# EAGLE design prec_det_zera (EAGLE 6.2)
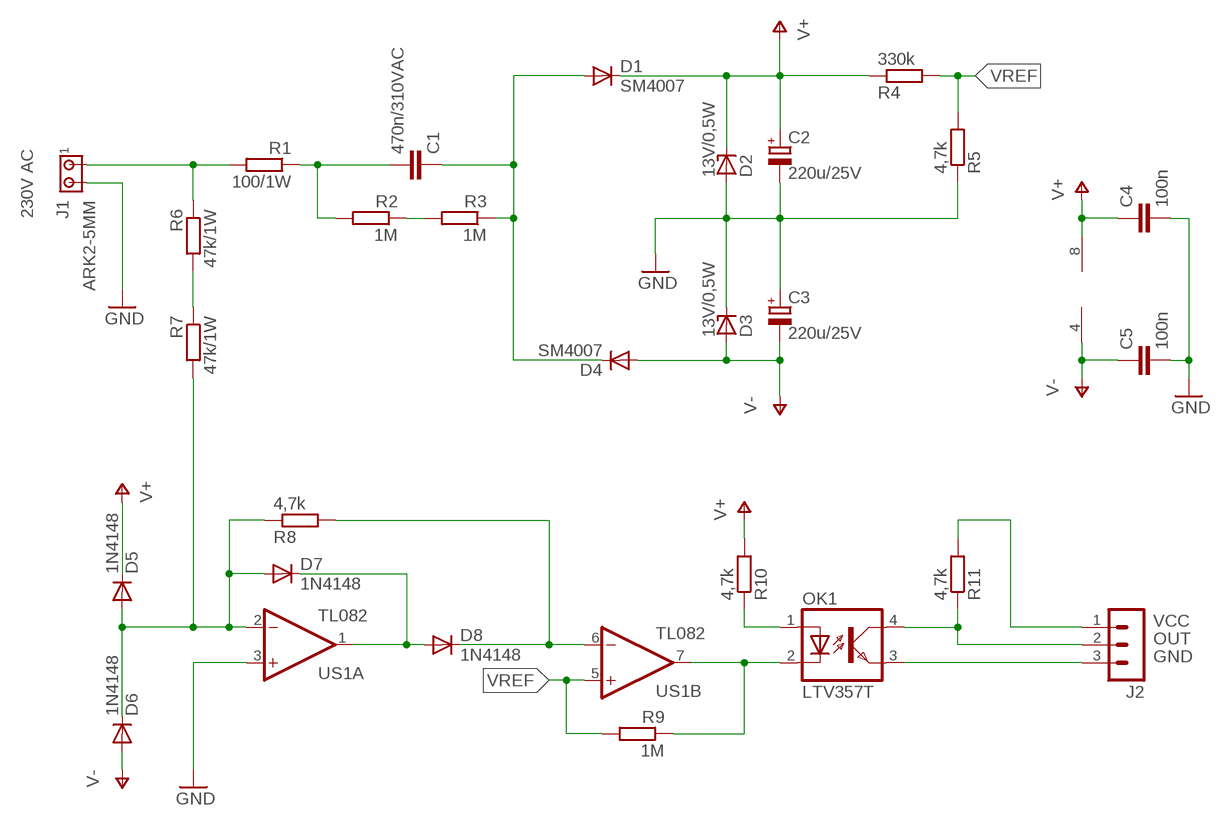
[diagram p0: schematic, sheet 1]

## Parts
C1  470n/310VAC  C-EU225-108X268  [C225-108X268]
C2  220u/25V  CPOL-EUE3.5-8  [E3,5-8]
C3  220u/25V  CPOL-EUE3.5-8  [E3,5-8]
C4  100n  C-EUC0805  [C0805]
C5  100n  C-EUC0805  [C0805]
D1  SM4007  DIODE-MELF-MLL41  [MELF-MLL41]
D2  13V/0,5W  ZENER-DIODESOD80C  [SOD80C]
D3  13V/0,5W  ZENER-DIODESOD80C  [SOD80C]
D4  SM4007  DIODE-MELF-MLL41  [MELF-MLL41]
D5  1N4148  DIODE-MINIMELF  [MINIMELF]
D6  1N4148  DIODE-MINIMELF  [MINIMELF]
D7  1N4148  DIODE-MINIMELF  [MINIMELF]
D8  1N4148  DIODE-MINIMELF  [MINIMELF]
J1  ARK2-5MM  [2PIN-5MM]
J2  MA03-1  [MA03-1]
OK1  LTV357T  SFH6186-3  [SMD4-7]
R1  100/1W  R-EU_0411/12  [0411/12]
R2  1M  R-EU_M0805  [M0805]
R3  1M  R-EU_M0805  [M0805]
R4  330k  R-EU_M0805  [M0805]
R5  4,7k  R-EU_M0805  [M0805]
R6  47k/1W  R-EU_0411/12  [0411/12]
R7  47k/1W  R-EU_0411/12  [0411/12]
R8  4,7k  R-EU_M0805  [M0805]
R9  1M  R-EU_M0805  [M0805]
R10  4,7k  R-EU_M0805  [M0805]
R11  4,7k  R-EU_M0805  [M0805]
US1  TL082  TL082D  [SO08]

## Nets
+15V: C2.+ C4.1 D1.C D2.C D5.C R4.1 R10.2 US1.8(P:V+) ; supply symbol labelled V+
-15V: C3.- C5.1 D3.A D4.A D6.A US1.4(P:V-) ; supply symbol labelled V-
GND: C2.- C3.+ C4.2 C5.2 D2.A D3.C J1.P$2 R5.1 US1.3(A:+IN)
N$1: OK1.2(C) R9.1 US1.7(B:OUT)
N$2: D5.A D6.C D7.A R7.2 R8.1 US1.2(A:-IN)
N$3: R6.2 R7.1
N$4: D7.C D8.A US1.1(A:OUT)
N$5: D8.C R8.2 US1.6(B:-IN)
N$6: OK1.1(A) R10.1
N$7: J2.3 OK1.3(EMIT)
N$8: J1.P$1 R1.2 R6.1
N$9: J2.2 OK1.4(COL) R11.1
N$10: J2.1 R11.2
N$17: C1.2 R1.1 R2.2
N$19: R2.1 R3.2
N$20: C1.1 D1.A D4.C R3.1
VREF: R4.2 R5.2 R9.2 US1.5(B:+IN)

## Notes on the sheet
- 230V AC
- VCC
- OUT
- GND

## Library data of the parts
C1 C4 C5 = rcl:C-EU: CAPACITOR, European symbol
C2 C3 = rcl:CPOL-EU: POLARIZED CAPACITOR, European symbol
D1 D4-D8 = diode:DIODE-: DIODE
D2 D3 = diode:ZENER-DIODE: Z-Diode
J1 = zlacza_futrzak:ARK2: ARK 2
J2 = con-lstb:MA03-1: PIN HEADER; OC_FARNELL: unknown; OC_NEWARK: unknown
OK1 = optocoupler:SFH618?*: Optocoupler, Phototransistor Output, Low Input Current Source: Data sheet; MF: VISHAY/TELEFUNKEN; MPN: SFH6186-3; OC_FARNELL: 1469529; OC_NEWARK: 21H7751
R1-R11 = rcl:R-EU_: RESISTOR, European symbol
US1 = linear:TL082: OP AMP

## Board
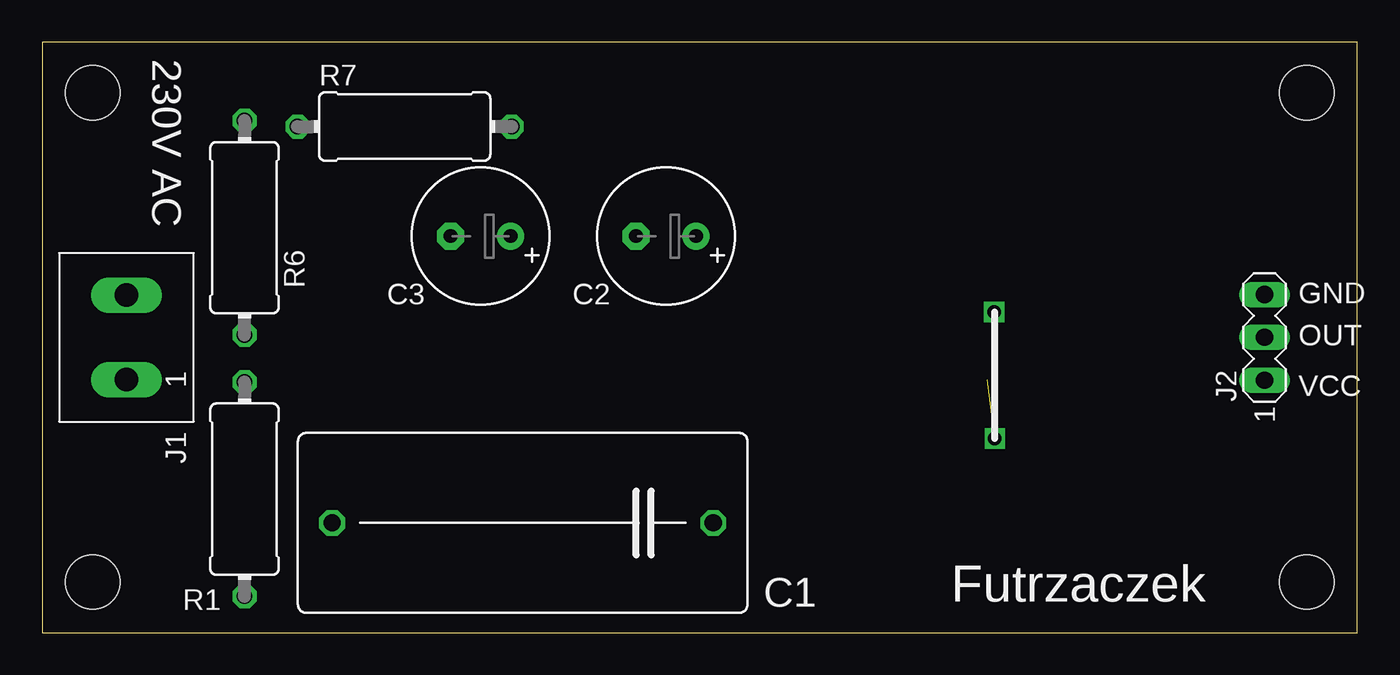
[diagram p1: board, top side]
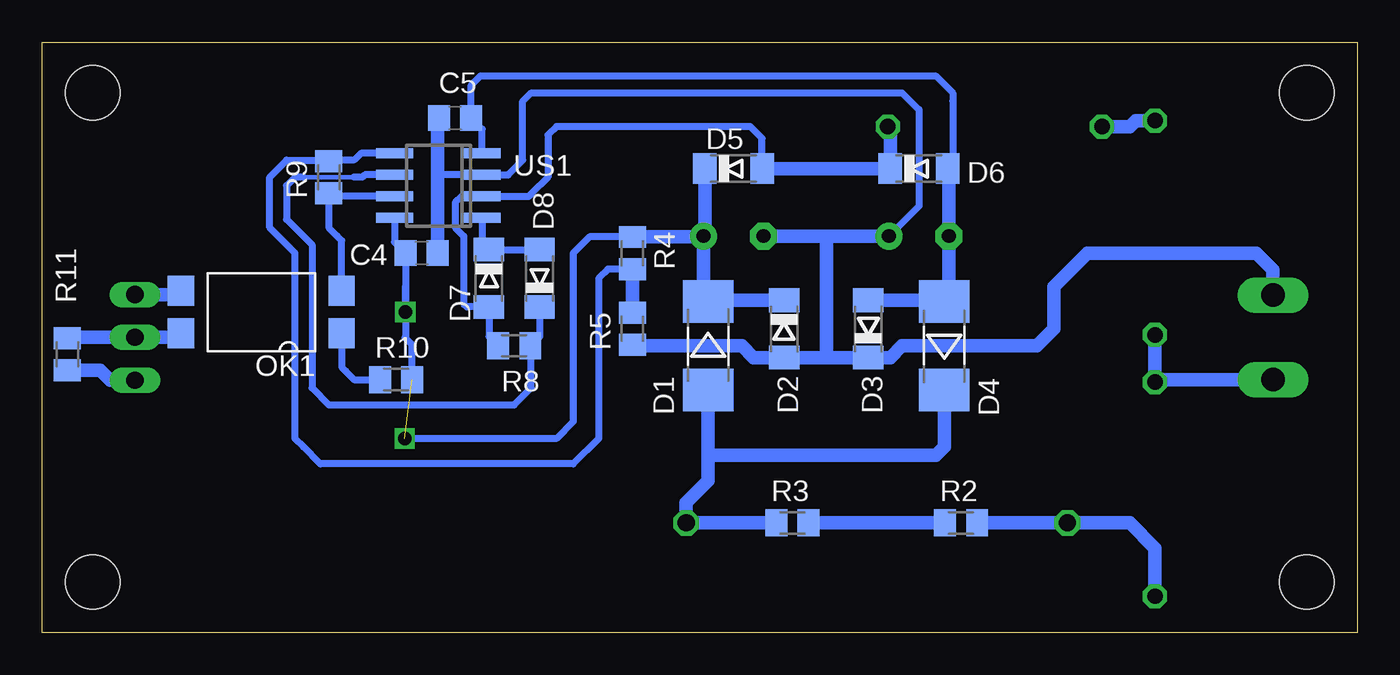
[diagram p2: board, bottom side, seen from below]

Size 78 x 35 mm. Coordinates in mm from the lower left corner, seen from the top.
Outline: 0,0 78,0 78,35 0,35 0,0
Copper layers (1*16): Top 0.035mm / dielectric 1.5mm / Bottom 0.035mm
Design rules: minimum track width 10mil, minimum drill 24mil, track to track 8mil, track to pad 8mil, pad to pad 8mil, via to via 8mil, smd to smd 8mil, copper to edge 40mil, drill to drill 8mil, minimum pad ring 10mil, minimum via ring 8mil, stop-mask expansion 4mil, vias tented up to drill 0mil, thermal gap 10mil
Holes 3.2 mm at 3,3 3,32 75,3 75,32

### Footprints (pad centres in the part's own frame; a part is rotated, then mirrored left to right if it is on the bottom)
C225-108X268 = drill 1.016 octagon: 1 -11.303,0; 2 11.303,0
E3,5-8 = drill 0.813 pad 1.6: + -1.778,0 | drill 0.813 pad 1.6 octagon: - 1.778,0
C0805 = smd 1.3 x 1.5: 1 -0.95,0; 2 0.95,0
MELF-MLL41 = smd 2.5 x 3: A 2.625,0; C -2.625,0
SOD80C = smd 1.4 x 1.8: A 1.7,0; C -1.7,0
MINIMELF = smd 1.4 x 1.8: A 1.7,0; C -1.7,0
2PIN-5MM = drill 1.4 long: P$1 -2.5,0; P$2 2.5,0
MA03-1 = drill 1.016 long: 1 -2.54,0; 2 0,0; 3 2.54,0
SMD4-7 = smd 1.78 x 1.55: 1 -1.27,-4.77; 2 1.27,-4.77; 3 1.27,4.77; 4 -1.27,4.77
0411/12 = drill 0.914 octagon: 1 -6.35,0; 2 6.35,0
M0805 = smd 1.3 x 1.6: 1 -0.95,0; 2 0.95,0
SO08 = smd 0.6 x 2.2: 1 -1.905,-2.6; 2 -0.635,-2.6; 3 0.635,-2.6; 4 1.905,-2.6; 5 1.905,2.6; 6 0.635,2.6; 7 -0.635,2.6; 8 -1.905,2.6

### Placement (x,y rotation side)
C1  28.5,6.5 180 top
C2  37,23.5 180 top
C3  26,23.5 180 top
C4  55.5,22.5 0 bottom
C5  53.5,30.5 180 bottom
D1  38.5,17 270 bottom
D2  34,18 270 bottom
D3  29,18 90 bottom
D4  24.5,17 90 bottom
D5  37,27.5 0 bottom
D6  26,27.5 0 bottom
D7  51.5,21 270 bottom
D8  48.5,21 90 bottom
J1  5,17.5 90 top
J2  72.5,17.5 90 top
OK1  65,19 90 bottom
R1  12,8.5 90 top
R2  23.5,6.5 0 bottom
R3  33.5,6.5 0 bottom
R4  43,22.5 270 bottom
R5  43,18 90 bottom
R6  12,24 90 top
R7  21.5,30 0 top
R8  50,17 0 bottom
R9  61,27 90 bottom
R10  57,15 0 bottom
R11  76.5,16.5 270 bottom
US1  54.5,26.5 90 bottom

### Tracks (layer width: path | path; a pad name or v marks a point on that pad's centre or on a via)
+15V  (via drill 0.8)  (1 unrouted)
  Bottom 0.406: US1.8 57.1,23.15 C4.1 56.45,20.5 | 56.45,20.5 v56.45,19 | v56.45,19 56.45,17.55 56.5,17.5 56.05,17.05 R10.2 | R4.1 45.55,23.45 46.5,22.5 46.5,12.5 47.5,11.5 v56.5,11.5 | v56.45,19 56.45,20.5
  Bottom 0.813: D2.C 38.42,19.7 D1.C 38.78,19.9 C2.+ | D5.C 38.7,23.58 C2.+ | R4.1 38.83,23.45 C2.+
-15V
  Bottom 0.406: D6.A 24,27.8 24,31.5 24,32 25,33 52,33 52.55,32.45 C5.1 51.9,29.85 US1.4
  Bottom 0.813: D3.A 24.57,19.7 D4.A 24.22,19.9 C3.- 24.22,27.92 D6.A
GND
  Bottom 0.406: 54.55,27 54.41,27.14 US1.3 50.37,27.14 50,27.5 49.5,28 49.5,31.5 49,32 27,32 26,31 26,25.28 C3.+
  Bottom 0.813: 31.5,16.3 D2.A 35.8,16.3 36.5,17 42.95,17 R5.1 | 31.5,16.3 D3.C 27.7,16.3 27,17 20,17 19,17 18,18 18,20.5 16,22.5 6,22.5 5,21.5 J1.P$2 | C3.+ 31,23.5 31.5,23.5 | 31.5,23.5 31.5,16.3 | C2.- 31.5,23.5 | C4.2 54.55,27 54.55,30.4 C5.2
N$1
  Bottom 0.406: US1.7 60.81,25.86 R9.1 61,24 60.5,23.5 60.23,23.23 OK1.2
N$2
  Bottom 0.406: R8.1 51.5,17.55 D7.A 52.8,19.3 53,19.5 53,23.5 53.5,24 53.5,25.5 53.13,25.86 US1.2 49.13,25.86 49,26 48,27 48,29.5 47.5,30 36,30 35.3,29.3 D5.A
  Bottom 0.813: D5.A D6.C 27.7,29.85 R7.2
N$3
  Bottom 0.813: R6.2 13.15,30.35 13.5,30 R7.1
N$4
  Bottom 0.406: US1.1 51.9,23.1 D7.C D8.A
N$5
  Bottom 0.254: 59.5,27 62.5,27
  Bottom 0.406: D8.C 48.5,17.55 R8.2 49,16.95 49,14.5 50,13.5 61,13.5 62,14.5 62,15.5 62,23 63.5,24.5 63.5,26.5 63,27 62.5,27 | US1.6 58.87,27.14 59,27 59.5,27
N$6
  Bottom 0.406: R10.1 59.5,15 60,15.5 60.23,15.73 OK1.1
N$7
  Bottom 0.813: J2.3 69.73,20.04 OK1.3
N$8
  Bottom 0.813: J1.P$1 11.85,15 R1.2 R6.1
N$9
  Bottom 0.813: OK1.4 69.73,17.5 J2.2 76.45,17.5 R11.1
N$10
  Bottom 0.813: R11.2 74.55,15.55 74.5,15.5 73.96,14.96 J2.1
N$17
  Bottom 0.813: R1.1 12,5 13.5,6.5 C1.2 R2.2
N$19
  Bottom 0.813: R2.1 R3.2
N$20
  Bottom 0.813: R3.1 C1.1 39.8,7.7 38.5,9 38.5,10.5 | D4.C 24.5,11 25,10.5 37.5,10.5 38.5,10.5 | 38.5,10.5 D1.A
VREF
  Bottom 0.406: US1.5 59.09,28.41 59.5,28 60.95,28 R9.2 61.05,28 63.5,28 64.5,27 64.5,24 63,22.5 63,11.5 62.5,11 61.5,10 46.5,10 45,11.5 45,21 44.45,21.55 R4.2
  Bottom 0.813: R4.2 R5.2

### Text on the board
tPlace: 230V AC | GND | OUT | VCC | Futrzaczek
